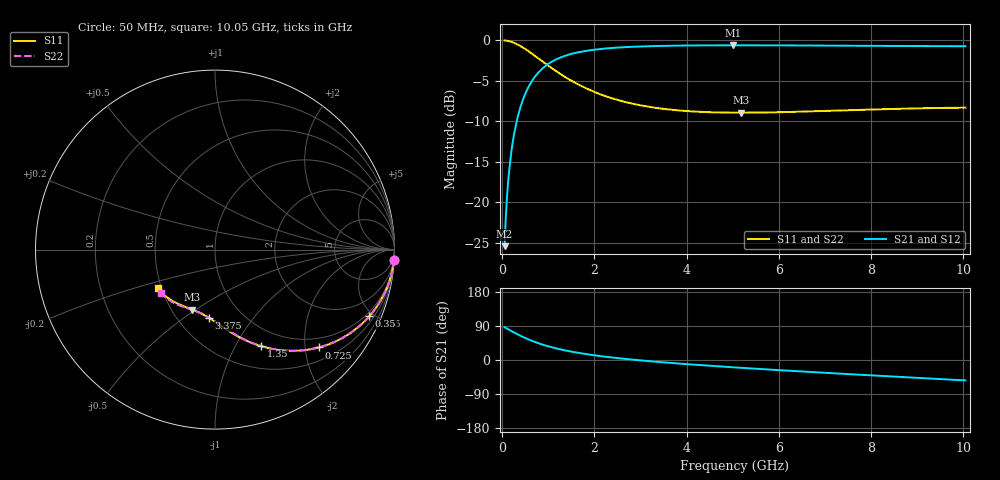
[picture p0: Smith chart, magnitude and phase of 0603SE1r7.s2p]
! AVX Thin Film Operation		Date: August 2001
! Description: Accu-P® Series, Thin Film, SMD, RF Capacitor
! Part Number: 06035J1R7ABT
! 50 MHz  -  10.05 GHz
! Serial Measurements
# mhz S db R 50
!	S11		S21		S12		S22
!	dB	Phase	dB	Phase	dB	Phase	dB	Phase
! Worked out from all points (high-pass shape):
!   401 points, 50 MHz to 10.05 GHz, reference 50 ohm
!   highest |S21| = -0.61 dB at 5 GHz (marker M1); lowest = -25.4 dB at 50 MHz (marker M2)
!   |S21| within 3 dB of the highest: 845.2 MHz to end of sweep
!   lowest |S11| = -8.9 dB at 5.175 GHz (marker M3), VSWR 2.11, Z = 31.5 - j24.2 ohm
!   |S11| at or under -10 dB: nowhere
!   |S22| runs from -8.9 to 0.0 dB; largest |S21 - S12| = 0
!   S11 on the Smith chart (normalised r, x): 50 MHz: 1, -33; 350 MHz: 0.78, -4.71; 725 MHz: 0.77, -2.30; 1.35 GHz: 0.77, -1.28; 3.375 GHz: 0.70, -0.63; 10.05 GHz: 0.48, -0.24
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50  -0.01 -3.5  -25.40 86.5  -25.40 86.5  -0.01 -3.5
75  -0.03 -5.2  -21.91 84.8  -21.91 84.8  -0.03 -5.2
125  -0.08 -8.7  -17.52 81.3  -17.52 81.3  -0.08 -8.7
175  -0.15 -12.0  -14.73 78.0  -14.73 78.0  -0.15 -12.0
250  -0.30 -17.0  -11.73 72.9  -11.73 72.9  -0.30 -17.0
350  -0.57 -23.4  -9.12 66.6  -9.12 66.6  -0.57 -23.4
425  -0.81 -27.8  -7.70 62.2  -7.70 62.2  -0.81 -27.8
525  -1.18 -33.4  -6.26 56.6  -6.26 56.6  -1.18 -33.4
725  -1.98 -43.2  -4.36 46.8  -4.36 46.8  -1.98 -43.2
1025  -3.24 -54.9  -2.79 35.1  -2.79 35.1  -3.24 -54.9
1350  -4.48 -64.3  -1.93 25.6  -1.93 25.6  -4.48 -64.3
1725  -5.66 -72.6  -1.39 17.4  -1.39 17.4  -5.65 -72.5
2050  -6.49 -78.5  -1.11 11.5  -1.11 11.5  -6.49 -78.3
2425  -7.23 -84.1  -0.92 6.0  -0.92 6.0  -7.23 -83.7
3375  -8.37 -95.2  -0.69 -5.0  -0.69 -5.0  -8.37 -94.5
3400  -8.39 -95.5  -0.69 -5.3  -0.69 -5.3  -8.38 -94.8
5000  -8.92 -110.0  -0.61 -19.2  -0.61 -19.2  -8.91 -108.3
5050  -8.92 -110.0  -0.61 -19.6  -0.61 -19.6  -8.91 -109.0
5175  -8.93 -110.9  -0.61 -20.6  -0.61 -20.6  -8.91 -109.9
6725  -8.77 -123.0  -0.64 -31.8  -0.64 -31.8  -8.74 -120.0
8400  -8.48 -135.1  -0.69 -43.2  -0.69 -43.2  -8.45 -131.1
10050  -8.31 -145.8  -0.72 -53.7  -0.72 -53.7  -8.28 -140.8
